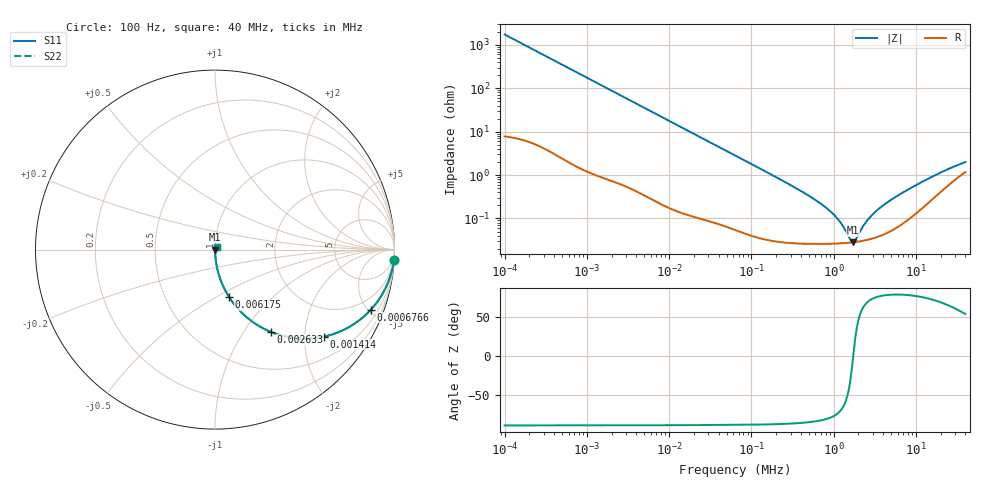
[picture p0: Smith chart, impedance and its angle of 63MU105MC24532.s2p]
!Components F PML CAP
!CONCATENATE F 0.1-40000kHz, at 20deg DC=0V
!Part Number F 63MU105MC24532
!Copyright(C) Rubycon Corporation. 20160805
# MHz S MA R 50
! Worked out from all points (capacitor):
!   561 points, 100 Hz to 40 MHz, reference 50 ohm
!   read as one part in series: C = 916 nF near 104.7 Hz
!   lowest |Z| = 28.4 mohm at 1.704 MHz (marker M1)
!   series resonance near 1.731 MHz, so ESL is about 9.2 nH
!   S11 on the Smith chart (normalised r, x): 100 Hz: 1, -35; 676.6 Hz: 1.03, -5.18; 1.414 kHz: 1.02, -2.48; 2.633 kHz: 1.01, -1.34; 6.175 kHz: 1.01, -0.57; 40 MHz: 1.02, +0.03
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0.0001  0.9981 -3.3  0.05749 86.4  0.05749 86.4  0.9981 -3.3
0.0002755255  0.9867 -9.0  0.1558 80.6  0.1558 80.6  0.9867 -9.0
0.0006765584  0.9308 -21.1  0.3594 68.6  0.3594 68.6  0.9308 -21.1
0.0008716573  0.8931 -26.4  0.4439 63.3  0.4439 63.3  0.8931 -26.4
0.001413914  0.7762 -38.7  0.6248 50.9  0.6248 50.9  0.7762 -38.7
0.002633433  0.5538 -55.9  0.8277 33.6  0.8277 33.6  0.5538 -55.9
0.003986471  0.4038 -65.6  0.911 23.8  0.911 23.8  0.4038 -65.6
0.006175306  0.2751 -73.5  0.9588 16.0  0.9588 16.0  0.2751 -73.5
0.007424854  0.2319 -76.0  0.9705 13.4  0.9705 13.4  0.2319 -76.0
0.01865671  0.09491 -83.9  0.9944 5.4  0.9944 5.4  0.09491 -83.9
0.06324555  0.02839 -87.3  0.9991 1.6  0.9991 1.6  0.02839 -87.3
0.5512845  0.002964 -84.8  0.9997 0.2  0.9997 0.2  0.002964 -84.8
1.0507  0.00112 -76.3  0.9997 0.1  0.9997 0.1  0.00112 -76.3
1.263305  0.0007216 -68.1  0.9997 0.0  0.9997 0.0  0.0007216 -68.1
1.590541  0.0003293 -32.5  0.9997 0.0  0.9997 0.0  0.0003293 -32.5
1.704339  0.0002835 -6.5  0.9997 0.0  0.9997 0.0  0.0002835 -6.5
1.826279  0.0003075 21.4  0.9997 -0.0  0.9997 -0.0  0.0003075 21.4
2.299343  0.0006756 63.0  0.9997 -0.0  0.9997 -0.0  0.0006756 63.0
2.764606  0.001067 71.8  0.9997 -0.1  0.9997 -0.1  0.001067 71.8
4.69589  0.002485 78.6  0.9995 -0.1  0.9995 -0.1  0.002485 78.6
14.51771  0.008442 73.3  0.9976 -0.5  0.9976 -0.5  0.008442 73.3
40  0.01965 53.1  0.9883 -0.9  0.9883 -0.9  0.01965 53.1
